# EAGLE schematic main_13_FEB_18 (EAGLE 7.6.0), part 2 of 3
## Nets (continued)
U_TRAP_2: IC159.15(D4)
U_TRAP_3: IC142.15(D4)
U_TRAP_4: IC129.15(D4)
U_TRAP_5: IC73.15(D4)
U_TRAP_6: IC34.15(D4)
U_TRAP_7: IC35.15(D4)
U_TRAP_8: IC36.15(D4)
U_TRAP_9: IC37.15(D4)
U_TRAP_10: IC38.15(D4)
U_TRAP_11: IC40.15(D4)
U_TRAP_12: IC41.15(D4)
U_TRAP_13: IC71.15(D4)
U_TRAP_14: IC20.15(D4)
U_TRAP_15: IC172.15(D4)
U_ZF: IC47.1(A:I0) IC126.2(1Q) IC127.2(A:I1) IC155.5(1C1)
U_ZF_IN_SRC: IC121.1(!A!/B)
UZF_AND_ALUZF: IC47.2(A:I1) IC119.3(B:I)
VCC: IC8.2(A:D) IC8.4(A:PRE) IC44.1(A:CLR) IC49.2(1A) IC56.5(1C1) IC163.2(A:D) IC163.4(A:PRE) IC164.2(A:D) IC164.4(A:PRE) IC168.2(A:D) IC168.4(A:PRE) IC174.2(A:D) IC174.4(A:PRE) IC187.2(A:D) IC187.4(A:PRE) IC188.2(A:D) IC188.4(A:PRE) IC204.4(A:PRE) IC221.2(A:D) IC221.4(A:PRE) IC222.6(G1) R1.2 R2.2 R3.2 R9.2
WR: IC60.5(Q2) IC69.13(B:A2)
XBUS0: IC2.18(Y1) IC9.18(Y1) IC25.9(B:Y1) IC27.9(B:Y1) IC103.18(Y1) IC104.18(Y1) IC105.9(B:Y1) IC107.9(B:Y1) IC109.9(B:Y1) IC111.9(B:Y1) IC113.18(Y1) IC114.18(Y1) IC116.18(Y1) IC117.18(Y1) IC122.18(Y1) IC125.18(Y1) IC140.18(Y1) IC145.18(Y1) IC154.18(Y1) IC181.18(A:Y1) IC210.18(Y1) IC244.9(B:Y1) IC245.18(Y1) RN1.1
XBUS1: IC2.17(Y2) IC9.17(Y2) IC25.7(B:Y2) IC27.7(B:Y2) IC105.7(B:Y2) IC107.7(B:Y2) IC109.7(B:Y2) IC111.7(B:Y2) IC113.17(Y2) IC114.17(Y2) IC116.17(Y2) IC117.17(Y2) IC122.17(Y2) IC125.17(Y2) IC145.17(Y2) IC154.17(Y2) IC181.16(A:Y2) IC245.17(Y2) RN1.2
XBUS2: IC2.16(Y3) IC9.16(Y3) IC25.5(B:Y3) IC27.5(B:Y3) IC105.5(B:Y3) IC107.5(B:Y3) IC109.5(B:Y3) IC111.5(B:Y3) IC113.16(Y3) IC114.16(Y3) IC116.16(Y3) IC117.16(Y3) IC122.16(Y3) IC125.16(Y3) IC145.16(Y3) IC154.16(Y3) IC181.14(A:Y3) IC245.16(Y3) RN1.3
XBUS3: IC2.15(Y4) IC9.15(Y4) IC25.3(B:Y4) IC27.3(B:Y4) IC105.3(B:Y4) IC107.3(B:Y4) IC109.3(B:Y4) IC111.3(B:Y4) IC113.15(Y4) IC114.15(Y4) IC116.15(Y4) IC117.15(Y4) IC122.15(Y4) IC125.15(Y4) IC145.15(Y4) IC154.15(Y4) IC181.12(A:Y4) IC244.3(B:Y4) IC245.15(Y4) RN1.4
XBUS4: IC24.9(B:Y1) IC26.9(B:Y1) IC106.9(B:Y1) IC108.9(B:Y1) IC110.9(B:Y1) IC112.9(B:Y1) IC116.14(Y5) IC125.14(Y5) IC154.14(Y5) IC176.18(A:Y1) IC245.14(Y5) IC247.9(B:Y1) RN1.5
XBUS5: IC24.7(B:Y2) IC26.7(B:Y2) IC106.7(B:Y2) IC108.7(B:Y2) IC110.7(B:Y2) IC112.7(B:Y2) IC116.13(Y6) IC125.13(Y6) IC154.13(Y6) IC176.16(A:Y2) IC245.13(Y6) RN1.6
XBUS6: IC24.5(B:Y3) IC26.5(B:Y3) IC106.5(B:Y3) IC108.5(B:Y3) IC110.5(B:Y3) IC112.5(B:Y3) IC113.12(Y7) IC114.12(Y7) IC115.12(Y7) IC116.12(Y7) IC125.12(Y7) IC154.12(Y7) IC176.14(A:Y3) IC245.12(Y7) RN1.7
XBUS7: IC2.11(Y8) IC3.11(Y8) IC9.11(Y8) IC24.3(B:Y4) IC26.3(B:Y4) IC80.4(B:I0) IC102.11(Y8) IC103.11(Y8) IC104.11(Y8) IC106.3(B:Y4) IC108.3(B:Y4) IC110.3(B:Y4) IC112.3(B:Y4) IC113.11(Y8) IC114.11(Y8) IC115.11(Y8) IC116.11(Y8) IC117.11(Y8) IC122.11(Y8) IC125.11(Y8) IC130.5(B:I1) IC140.11(Y8) IC145.11(Y8) IC146.11(Y8) IC154.11(Y8) IC176.12(A:Y4) IC210.11(Y8) IC245.11(Y8) IC247.3(B:Y4) RN1.8
XBUS8: IC146.18(Y1)
XBUS9: IC146.17(Y2)
XBUS10: IC146.16(Y3)
XBUS11: IC146.15(Y4)
XBUS12: IC171.18(Y1) IC215.18(Y1)
XBUS13: IC171.11(Y8) IC215.11(Y8)
XBUS14: IC259.18(Y1) IC260.18(Y1)
XBUS15: IC259.11(Y8) IC260.11(Y8)
XBUS16: IC89.18(A:Y1) IC91.18(A:Y1)
XBUS17: IC89.16(A:Y2) IC91.16(A:Y2)
XBUS18: IC89.14(A:Y3) IC91.14(A:Y3)
XBUS19: IC89.12(A:Y4) IC91.12(A:Y4)
XBUS20: IC90.18(A:Y1) IC92.18(A:Y1)
XBUS21: IC90.16(A:Y2) IC92.16(A:Y2)
XBUS22: IC90.14(A:Y3) IC92.14(A:Y3)
XBUS23: IC90.12(A:Y4) IC92.12(A:Y4)
XBUS24: IC14.1(B0) RN2.1
XBUS25: IC14.22(B1) RN2.2
XBUS26: IC14.20(B2) RN2.3
XBUS27: IC14.18(B3) RN2.4
XBUS28: IC11.12(A:Y4) IC15.1(B0) RN2.5
XBUS29: IC11.14(A:Y3) IC15.22(B1) RN2.6
XBUS30: IC11.16(A:Y2) IC15.20(B2) RN2.7
XBUS31: IC11.18(A:Y1) IC15.18(B3) RN2.8
XBUS32: IC102.18(Y1)
XBUS33: IC102.17(Y2)
XBUS34: IC102.16(Y3)
XBUS35: IC102.15(Y4)
XBUS36: IC263.18(Y1) IC264.18(Y1)
XBUS37: IC263.11(Y8) IC264.11(Y8)
XBUS38: IC252.18(Y1) IC253.18(Y1)
XBUS39: IC252.11(Y8) IC253.11(Y8)
XBUS40: IC3.18(Y1)
XBUS41: IC3.17(Y2)
XBUS42: IC3.16(Y3)
XBUS43: IC3.15(Y4)
XBUS44: IC266.18(Y1) IC267.18(Y1)
XBUS45: IC266.11(Y8) IC267.11(Y8)
XBUS46: IC298.18(A:Y1)
XBUS47: IC298.16(A:Y2)
XBUS48: IC115.18(Y1)
XBUS49: IC115.17(Y2)
XBUS50: IC115.16(Y3)
XBUS51: IC115.15(Y4)
XBUS52: IC298.14(A:Y3)
XBUS53: IC298.12(A:Y4)
XBUS54: IC297.18(A:Y1)
XBUS55: IC297.16(A:Y2)
XBUS56: IC15.19(A3) RN3.1
XBUS57: IC15.21(A2) RN3.2
XBUS58: IC15.23(A1) RN3.3
XBUS59: IC15.2(A0) RN3.4
XBUS60: IC14.19(A3) RN3.5
XBUS61: IC14.21(A2) RN3.6
XBUS62: IC14.23(A1) RN3.7
XBUS63: IC14.2(A0) RN3.8
XBUS64: IC297.14(A:Y3)
XBUS65: IC297.12(A:Y4)
XBUS66: IC289.12(A:Y4)
XBUS67: IC289.14(A:Y3)
XBUS68: IC289.16(A:Y2)
XBUS69: IC289.18(A:Y1)
YBUS0: IC19.18(Y1) IC182.18(A:Y1)
YBUS1: IC19.17(Y2) IC182.16(A:Y2)
YBUS2: IC19.16(Y3) IC182.14(A:Y3)
YBUS3: IC19.15(Y4) IC182.12(A:Y4)
YBUS4: IC19.14(Y5) IC183.18(A:Y1)
YBUS5: IC183.16(A:Y2)
YBUS6: IC183.14(A:Y3)
YBUS7: IC19.11(Y8) IC130.4(B:I0) IC183.12(A:Y4)
YBUS8: IC299.18(A:Y1)
YBUS9: IC299.16(A:Y2)
YBUS10: IC299.14(A:Y3)
YBUS11: IC299.12(A:Y4)
YBUS12: IC300.18(A:Y1)
YBUS13: IC300.16(A:Y2)
YBUS14: IC300.14(A:Y3)
YBUS15: IC300.12(A:Y4)
YBUS16: IC211.18(A:Y1) IC213.18(A:Y1)
YBUS17: IC211.16(A:Y2) IC213.16(A:Y2)
YBUS18: IC211.14(A:Y3) IC213.14(A:Y3)
YBUS19: IC211.12(A:Y4) IC213.12(A:Y4)
YBUS20: IC212.18(A:Y1) IC214.18(A:Y1)
YBUS21: IC212.16(A:Y2) IC214.16(A:Y2)
YBUS22: IC212.14(A:Y3) IC214.14(A:Y3)
YBUS23: IC212.12(A:Y4) IC214.12(A:Y4)
YBUS40: IC229.18(A:Y1) IC231.18(A:Y1)
YBUS41: IC229.16(A:Y2) IC231.16(A:Y2)
YBUS42: IC229.14(A:Y3) IC231.14(A:Y3)
YBUS43: IC229.12(A:Y4) IC231.12(A:Y4)
YBUS44: IC230.18(A:Y1) IC232.18(A:Y1)
YBUS45: IC230.16(A:Y2) IC232.16(A:Y2)
YBUS46: IC230.14(A:Y3) IC232.14(A:Y3)
YBUS47: IC230.12(A:Y4) IC232.12(A:Y4)
YBUS48: IC235.18(A:Y1) IC237.18(A:Y1)
YBUS49: IC235.16(A:Y2) IC237.16(A:Y2)
YBUS50: IC235.14(A:Y3) IC237.14(A:Y3)
YBUS51: IC235.12(A:Y4) IC237.12(A:Y4)
YBUS52: IC236.18(A:Y1) IC238.18(A:Y1)
YBUS53: IC236.16(A:Y2) IC238.16(A:Y2)
YBUS54: IC236.14(A:Y3) IC238.14(A:Y3)
YBUS55: IC236.12(A:Y4) IC238.12(A:Y4)
ZBUFF0_16: IC86.3(1D) IC88.3(1D)
ZBUFF0_17: IC86.4(2D) IC88.4(2D)
ZBUFF0_18: IC86.7(3D) IC88.7(3D)
ZBUFF0_19: IC86.8(4D) IC88.8(4D)
ZBUFF0_20: IC86.13(5D) IC88.13(5D)
ZBUFF0_21: IC88.14(6D)
ZBUFF0_22: IC86.14(6D) IC86.17(7D) IC88.17(7D)
ZBUFF0_23: IC86.18(8D) IC88.18(8D)
ZBUFF0_24: IC16.3(1D) IC17.3(1D)
ZBUFF0_25: IC16.4(2D) IC17.4(2D)
ZBUFF0_26: IC16.7(3D) IC17.7(3D)
ZBUFF0_27: IC16.8(4D) IC17.8(4D)
ZBUFF0_28: IC16.13(5D) IC17.13(5D)
ZBUFF0_29: IC16.14(6D) IC17.14(6D)
ZBUFF0_30: IC16.17(7D) IC17.17(7D)
ZBUFF0_31: IC16.18(8D) IC17.18(8D)
ZBUFF0_56: IC233.3(1D) IC234.3(1D)
ZBUFF0_57: IC233.4(2D) IC234.4(2D)
ZBUFF0_58: IC233.7(3D) IC234.7(3D)
ZBUFF0_59: IC233.8(4D) IC234.8(4D)
ZBUFF0_60: IC233.13(5D) IC234.13(5D)
ZBUFF0_61: IC233.14(6D) IC234.14(6D)
ZBUFF0_62: IC233.17(7D) IC234.17(7D)
ZBUFF0_63: IC233.18(8D) IC234.18(8D)
ZBUFF0_64: IC239.3(1D) IC240.3(1D)
ZBUFF0_65: IC239.4(2D) IC240.4(2D)
ZBUFF0_66: IC239.7(3D) IC240.7(3D)
ZBUFF0_67: IC239.8(4D) IC240.8(4D)
ZBUFF0_68: IC239.13(5D) IC240.13(5D)
ZBUFF0_69: IC239.14(6D) IC240.14(6D)
ZBUFF0_70: IC239.17(7D) IC240.17(7D)
ZBUFF0_71: IC239.18(8D) IC240.18(8D)
ZBUFF1_0: IC4.3(1D) IC5.3(1D) IC98.3(1D) IC99.3(1D)
ZBUFF1_1: IC4.4(2D) IC5.4(2D) IC98.4(2D) IC99.4(2D)
ZBUFF1_2: IC4.7(3D) IC5.7(3D) IC98.7(3D) IC99.7(3D)
ZBUFF1_3: IC4.8(4D) IC5.8(4D) IC98.8(4D) IC99.8(4D)
ZBUFF1_4: IC4.13(5D) IC5.13(5D) IC98.13(5D) IC99.13(5D)
ZBUFF1_5: IC4.14(6D) IC5.14(6D) IC98.14(6D) IC99.14(6D)
ZBUFF1_6: IC4.17(7D) IC5.17(7D) IC98.17(7D) IC99.17(7D)
ZBUFF1_7: IC4.18(8D) IC5.18(8D) IC98.18(8D) IC99.18(8D)
ZBUFF1_8: IC173.3(1D) IC205.3(1D)
ZBUFF1_9: IC173.4(2D) IC205.4(2D)
ZBUFF1_10: IC173.7(3D) IC205.7(3D)
ZBUFF1_11: IC173.8(4D) IC205.8(4D)
ZBUFF1_12: IC173.13(5D) IC205.13(5D)
ZBUFF1_13: IC173.14(6D) IC205.14(6D)
ZBUFF1_14: IC173.17(7D) IC205.17(7D)
ZBUFF1_15: IC173.18(8D) IC205.18(8D)
ZBUFF1_16: IC165.3(1D) IC166.3(1D)
ZBUFF1_17: IC165.4(2D) IC166.4(2D)
ZBUFF1_18: IC165.7(3D) IC166.7(3D)
ZBUFF1_19: IC165.8(4D) IC166.8(4D)
ZBUFF1_20: IC165.13(5D) IC166.13(5D)
ZBUFF1_21: IC165.14(6D) IC166.14(6D)
ZBUFF1_22: IC165.17(7D) IC166.17(7D)
ZBUFF1_23: IC165.18(8D) IC166.18(8D)
ZBUFF1_24: IC217.3(1D) IC246.3(1D)
ZBUFF1_25: IC217.4(2D) IC246.4(2D)
ZBUFF1_26: IC217.7(3D) IC246.7(3D)
ZBUFF1_27: IC217.8(4D) IC246.8(4D)
ZBUFF1_28: IC217.13(5D) IC246.13(5D)
ZBUFF1_29: IC217.14(6D) IC246.14(6D)
ZBUFF1_30: IC217.17(7D) IC246.17(7D)
ZBUFF1_31: IC217.18(8D) IC246.18(8D)
ZBUFF1_32: IC261.3(1D) IC262.3(1D)
ZBUFF1_33: IC261.4(2D) IC262.4(2D)
ZBUFF1_34: IC261.7(3D) IC262.7(3D)
ZBUFF1_35: IC261.8(4D) IC262.8(4D)
ZBUFF1_36: IC261.13(5D) IC262.13(5D)
ZBUFF1_37: IC261.14(6D) IC262.14(6D)
ZBUFF1_38: IC261.17(7D) IC262.17(7D)
ZBUFF1_39: IC261.18(8D) IC262.18(8D)
ZBUFF1_40: IC202.3(1D) IC251.3(1D)
ZBUFF1_41: IC202.4(2D) IC251.4(2D)
ZBUFF1_42: IC202.7(3D) IC251.7(3D)
ZBUFF1_43: IC202.8(4D) IC251.8(4D)
ZBUFF1_44: IC202.13(5D) IC251.13(5D)
ZBUFF1_45: IC202.14(6D) IC251.14(6D)
ZBUFF1_46: IC202.17(7D) IC251.17(7D)
ZBUFF1_47: IC202.18(8D) IC251.18(8D)
ZBUFF1_48: IC254.3(1D) IC265.3(1D)
ZBUFF1_49: IC254.4(2D) IC265.4(2D)
ZBUFF1_50: IC254.7(3D) IC265.7(3D)
ZBUFF1_51: IC254.8(4D) IC265.8(4D)
ZBUFF1_52: IC254.13(5D) IC265.13(5D)
ZBUFF1_53: IC254.14(6D) IC265.14(6D)
ZBUFF1_54: IC254.17(7D) IC265.17(7D)
ZBUFF1_55: IC254.18(8D) IC265.18(8D)
ZBUFF2_0: IC1.3(1D) IC23.14(4A) IC100.3(1D) IC101.3(1D)
ZBUFF2_1: IC1.4(2D) IC23.11(3A) IC100.4(2D) IC101.4(2D)
ZBUFF2_2: IC1.7(3D) IC23.5(2A) IC100.7(3D) IC101.7(3D)
ZBUFF2_3: IC1.8(4D) IC23.2(1A) IC100.8(4D) IC101.8(4D)
ZBUFF2_4: IC1.13(5D) IC22.14(4A) IC100.13(5D) IC101.13(5D)
ZBUFF2_5: IC1.14(6D) IC22.11(3A) IC100.14(6D) IC101.14(6D)
ZBUFF2_6: IC1.17(7D) IC22.5(2A) IC100.17(7D) IC101.17(7D)
ZBUFF2_7: IC22.2(1A) IC100.18(8D) IC101.18(8D)
ZBUFF2_16: IC123.3(1D)
ZBUFF2_17: IC123.4(2D)
ZBUFF2_18: IC123.7(3D)
ZBUFF2_19: IC123.8(4D)
ZBUFF2_20: IC123.13(5D)
ZBUFF2_21: IC123.14(6D)
ZBUFF2_22: IC123.17(7D)
ZBUFF2_23: IC153.3(1D)
ZBUFF2_24: IC153.4(2D)
ZBUFF2_25: IC153.7(3D)
ZBUFF2_26: IC153.8(4D)
ZBUFF2_27: IC153.13(5D)
ZBUFF2_28: IC153.14(6D)
ZBUFF2_29: IC153.17(7D)
ZBUFF2_30: IC153.18(8D)
ZBUFF2_31: IC185.3(1D)
ZBUFF2_32: IC185.4(2D)
ZBUFF2_33: IC185.7(3D)
ZBUFF2_34: IC185.8(4D)
ZBUFF2_35: IC185.13(5D)
ZBUFF2_36: IC185.14(6D)
ZBUFF2_37: IC185.17(7D)
ZBUFF2_38: IC185.18(8D)
ZBUS0: IC6.3(1D) IC7.3(1D) IC48.3(1D) IC96.2(1A) IC97.2(1A) IC144.14(D1) IC175.4(B:I0) IC184.3(1D) IC189.3(1D) IC197.1(A:I0) IC216.3(1D) IC241.3(1C3) IC248.14(D1) RN5.1
ZBUS1: IC96.5(2A) IC97.5(2A) IC144.13(D2) IC175.5(B:I1) IC184.4(2D) IC197.2(A:I1) IC216.4(2D) IC243.3(1C3) IC248.13(D2) RN5.2
ZBUS2: IC96.11(3A) IC97.11(3A) IC144.12(D3) IC177.5(B:I1) IC184.7(3D) IC197.3(A:I2) IC216.7(3D) IC248.12(D3) IC255.3(1C3) RN5.3
ZBUS3: IC96.14(4A) IC97.14(4A) IC144.11(D4) IC184.8(4D) IC192.5(B:I1) IC197.12(A:I3) IC216.8(4D) IC248.11(D4) IC256.3(1C3) RN5.4
ZBUS4: IC94.2(1A) IC95.2(1A) IC128.14(D1) IC184.13(5D) IC193.5(B:I1) IC197.13(A:I4) IC208.3(1C3) IC216.13(5D) IC249.14(D1) RN5.5
ZBUS5: IC94.5(2A) IC95.5(2A) IC128.13(D2) IC184.14(6D) IC194.5(B:I1) IC199.2(A:I1) IC216.14(6D) IC249.13(D2) RN5.6
ZBUS6: IC94.11(3A) IC95.11(3A) IC128.12(D3) IC184.17(7D) IC199.3(A:I2) IC200.5(B:I1) IC216.17(7D) IC249.12(D3) RN5.7
ZBUS7: IC6.18(8D) IC7.18(8D) IC48.18(8D) IC80.5(B:I1) IC94.14(4A) IC95.14(4A) IC128.11(D4) IC184.18(8D) IC189.18(8D) IC199.12(A:I3) IC209.5(B:I1) IC216.18(8D) IC249.11(D4) IC255.5(1C1) RN5.8
ZF: IC120.2(A:I1) IC122.2(A1) IC155.6(1C0) IC227.2(Q1) IC241.6(1C0)
ZF_FROM_ALU: IC120.1(A:I0) IC121.2(1A) IC124.1(A:I0) IC127.1(A:I0) IC155.4(1C2) IC199.5(A:O) IC241.5(1C1)
ZF_IN_SRC_0: IC241.14(A)
ZF_IN_SRC_1: IC241.2(B)
~CLK: IC32.11(CLK) IC33.11(CLK)
~RST: IC32.1(CLR) IC33.1(CLR) IC44.4(A:PRE) IC54.4(B:O) IC162.1(CLR) IC195.1(A:I0) IC204.1(A:CLR) IC207.2(A:I1) IC218.1(A:I0) IC219.1(A:I0) IC220.2(A:I1) IC223.2(A:I1) IC224.2(A:I1) IC225.2(A:I1) IC227.1(CLR)
Unconnected: IC1.11(CLK) IC1.18(8D) IC2.12(Y7) IC2.13(Y6) IC2.14(Y5) IC3.12(Y7) IC3.13(Y6) IC3.14(Y5) IC4.11(CLK) IC5.11(CLK) IC6.4(2D) IC6.7(3D) IC6.8(4D) IC6.11(CLK) IC6.13(5D) IC6.14(6D) IC6.17(7D) IC7.4(2D) IC7.7(3D) IC7.8(4D) IC7.13(5D) IC7.14(6D) IC7.17(7D) IC8.6(A:!Q) IC8.8(B:!Q) IC8.9(B:Q) IC8.10(B:PRE) IC8.11(B:CLK) IC8.12(B:D) IC8.13(B:CLR) IC9.12(Y7) IC9.13(Y6) IC9.14(Y5) IC10.3(B:Y4) IC10.5(B:Y3) IC10.7(B:Y2) IC10.9(B:Y1) IC10.11(B:A1) IC10.13(B:A2) IC10.15(B:A3) IC10.17(B:A4) IC10.19(B:G) IC11.3(B:Y4) IC11.5(B:Y3) IC11.7(B:Y2) IC11.9(B:Y1) IC11.11(B:A1) IC11.13(B:A2) IC11.15(B:A3) IC11.17(B:A4) IC11.19(B:G) IC12.3(B:Y4) IC12.5(B:Y3) IC12.7(B:Y2) IC12.9(B:Y1) IC12.11(B:A1) IC12.13(B:A2) IC12.15(B:A3) IC12.17(B:A4) IC12.19(B:G) IC13.3(B:Y4) IC13.5(B:Y3) IC13.7(B:Y2) IC13.9(B:Y1) IC13.11(B:A1) IC13.13(B:A2) IC13.15(B:A3) IC13.17(B:A4) IC13.19(B:G) IC14.14(A=B) IC14.15(P) IC14.17(G) IC15.14(A=B) IC15.15(P) IC15.17(G) IC16.11(CLK) IC17.11(CLK) IC18.1(A:I0) IC18.2(A:I1) IC18.3(A:O) IC18.8(C:O) IC18.9(C:I0) IC18.10(C:I1) IC18.11(D:O) IC18.12(D:I0) IC18.13(D:I1) IC19.2(A1) IC19.3(A2) IC19.4(A3) IC19.5(A4) IC19.6(A5) IC19.7(A6) IC19.8(A7) IC19.9(A8) IC19.12(Y7) IC19.13(Y6) IC20.6(W) IC20.7(G) IC20.9(C) IC20.10(B) IC20.11(A) IC20.12(D7) IC20.13(D6) IC21.11(CLK) IC24.1(A:G) IC24.2(A:A1) IC24.4(A:A2) IC24.6(A:A3) IC24.8(A:A4) IC24.12(A:Y4) IC24.14(A:Y3) IC24.16(A:Y2) IC24.18(A:Y1) IC25.1(A:G) IC25.2(A:A1) IC25.4(A:A2) IC25.6(A:A3) IC25.8(A:A4) IC25.12(A:Y4) IC25.14(A:Y3) IC25.16(A:Y2) IC25.18(A:Y1) IC26.1(A:G) IC26.2(A:A1) IC26.4(A:A2) IC26.6(A:A3) IC26.8(A:A4) IC26.12(A:Y4) IC26.14(A:Y3) IC26.16(A:Y2) IC26.18(A:Y1) IC27.1(A:G) IC27.2(A:A1) IC27.4(A:A2) IC27.6(A:A3) IC27.8(A:A4) IC27.12(A:Y4) IC27.14(A:Y3) IC27.16(A:Y2) IC27.18(A:Y1) IC28.6(A5) IC28.7(A6) IC28.8(A7) IC28.9(A8) IC28.11(Y8) IC28.12(Y7) IC28.13(Y6) IC28.14(Y5) IC30.3(B:Y4) IC30.5(B:Y3) IC30.7(B:Y2) IC30.9(B:Y1) IC30.11(B:A1) IC30.13(B:A2) IC30.15(B:A3) IC30.17(B:A4) IC30.19(B:G) IC31.3(B:Y4) IC31.5(B:Y3) IC31.7(B:Y2) IC31.9(B:Y1) IC31.11(B:A1) IC31.13(B:A2) IC31.15(B:A3) IC31.17(B:A4) IC31.19(B:G) IC34.6(W) IC34.7(G) IC34.9(C) IC34.10(B) IC34.11(A) IC34.12(D7) IC34.13(D6) IC35.6(W) IC35.7(G) IC35.9(C) IC35.10(B) IC35.11(A) IC35.12(D7) IC35.13(D6) IC36.6(W) IC36.7(G) IC36.9(C) IC36.10(B) IC36.11(A) IC36.12(D7) IC36.13(D6) IC37.6(W) IC37.7(G) IC37.9(C) IC37.10(B) IC37.11(A) IC37.12(D7) IC37.13(D6) IC38.6(W) IC38.7(G) IC38.9(C) IC38.10(B) IC38.11(A) IC38.12(D7) IC38.13(D6) IC39.4(B:I0) IC39.5(B:I1) IC39.6(B:O) IC39.8(C:O) IC39.9(C:I0) IC39.10(C:I1) IC39.11(D:O) IC39.12(D:I0) IC39.13(D:I1) IC40.6(W) IC40.7(G) IC40.9(C) IC40.10(B) IC40.11(A) IC40.12(D7) IC40.13(D6) IC41.6(W) IC41.7(G) IC41.9(C) IC41.10(B) IC41.11(A) IC41.12(D7) IC41.13(D6) IC42.4(B:I0) IC42.5(B:I1) IC42.6(B:O) IC42.8(C:O) IC42.9(C:I0) IC42.10(C:I1) IC42.11(D:O) IC42.12(D:I0) IC42.13(D:I1) IC43.1(A:I) IC43.2(A:O) IC43.5(C:I) IC43.6(C:O) IC43.8(D:O) IC43.9(D:I) IC43.10(E:O) IC43.11(E:I) IC43.12(F:O) IC43.13(F:I) IC44.6(A:!Q) IC44.8(B:!Q) IC44.9(B:Q) IC44.10(B:PRE) IC44.11(B:CLK) IC44.12(B:D) IC44.13(B:CLR) IC45.4(B:I0) IC45.5(B:I1) IC45.6(B:O) IC45.8(C:O) IC45.9(C:I0) IC45.10(C:I1) IC45.11(D:O) IC45.12(D:I0) IC45.13(D:I1) IC46.1(A:I0) IC46.2(A:I1) IC46.3(A:O) IC46.8(C:O) IC46.9(C:I0) IC46.10(C:I1) IC46.11(D:O) IC46.12(D:I0) IC46.13(D:I1) IC47.4(B:I0) IC47.5(B:I1) IC47.6(B:O) IC47.8(C:O) IC47.9(C:I0) IC47.10(C:I1) IC47.11(D:O) IC47.12(D:I0) IC47.13(D:I1) IC48.4(2D) IC48.7(3D) IC48.8(4D) IC48.11(CLK) IC48.13(5D) IC48.14(6D) IC48.17(7D) IC50.1(S2) IC50.10(S4) IC50.13(S3) IC51.1(S2) IC51.4(S1) IC51.10(S4) IC51.13(S3) IC52.1(S2) IC52.4(S1) IC52.10(S4) IC52.13(S3) IC53.4(S1) IC53.9(C4) IC53.10(S4) IC53.13(S3) IC54.1(A:I) IC54.2(A:O) IC54.5(C:I) IC54.6(C:O) IC54.8(D:O) IC54.9(D:I) IC54.10(E:O) IC54.11(E:I) IC54.12(F:O) IC54.13(F:I) IC56.9(2Y) IC56.10(2C0) IC56.11(2C1) IC56.12(2C2) IC56.13(2C3) IC57.5(C:I) IC57.6(C:O) IC57.8(D:O) IC57.9(D:I) IC57.10(E:O) IC57.11(E:I) IC57.12(F:O) IC57.13(F:I) IC58.4(B:I0) IC58.5(B:I1) IC58.6(B:O) IC58.8(C:O) IC58.9(C:I0) IC58.10(C:I1) IC58.11(D:O) IC58.12(D:I0) IC58.13(D:I1) IC59.3(B:I) IC59.4(B:O) IC59.5(C:I) IC59.6(C:O) IC59.8(D:O) IC59.9(D:I) IC59.10(E:O) IC59.11(E:I) IC59.12(F:O) IC59.13(F:I) IC60.1(CLR) IC60.9(Q4) IC60.12(Q5) IC60.15(Q6) IC60.16(Q7) IC60.19(Q8) IC61.1(CLR) IC61.2(Q1) IC61.5(Q2) IC61.6(Q3) IC61.9(Q4) IC61.12(Q5) IC61.15(Q6) IC61.16(Q7) IC61.19(Q8) IC62.1(CLR) IC62.2(Q1) IC62.5(Q2) IC62.6(Q3) IC62.9(Q4) IC62.12(Q5) IC62.15(Q6) IC62.16(Q7) IC62.19(Q8) IC64.3(B:I0) IC64.4(B:I1) IC64.5(B:I2) IC64.6(B:O) IC64.8(C:O) IC64.9(C:I0) IC64.10(C:I1) IC64.11(C:I2) IC65.4(B:O) IC65.5(B:I0) IC65.6(B:I1) IC65.8(C:I0) IC65.9(C:I1) IC65.10(C:O) IC65.11(D:I0) IC65.12(D:I1) IC65.13(D:O) IC66.4(B:O) IC66.5(B:I0) IC66.6(B:I1) IC66.8(C:I0) IC66.9(C:I1) IC66.10(C:O) IC66.11(D:I0) IC66.12(D:I1) IC66.13(D:O) IC67.1(A:I0) IC67.2(A:I1) IC67.3(A:O) IC67.8(C:O) IC67.9(C:I0) IC67.10(C:I1) IC67.11(D:O) IC67.12(D:I0) IC67.13(D:I1) IC68.9(3Y) IC68.12(4Y) IC69.1(A:G) IC69.2(A:A1) IC69.3(B:Y4) IC69.4(A:A2) IC69.6(A:A3) IC69.8(A:A4) IC69.12(A:Y4) IC69.14(A:Y3) IC69.16(A:Y2) IC69.18(A:Y1) IC70.6(W) IC71.6(W) IC71.7(G) IC71.9(C) IC71.10(B) IC71.11(A) IC71.12(D7) IC71.13(D6) IC72.1(A:I0) IC72.2(A:I1) IC72.3(A:O) IC72.8(C:O) IC72.9(C:I0) IC72.10(C:I1) IC72.11(D:O) IC72.12(D:I0) IC72.13(D:I1) IC73.6(W) IC73.7(G) IC73.9(C) IC73.10(B) IC73.11(A) IC73.12(D7) IC73.13(D6) IC74.1(A:I0) IC74.2(A:I1) IC74.3(A:O) IC74.8(C:O) IC74.9(C:I0) IC74.10(C:I1) IC74.11(D:O) IC74.12(D:I0) IC74.13(D:I1) IC75.2(Q1) IC75.5(Q2) IC75.6(Q3) IC75.9(Q4) IC75.12(Q5) IC75.15(Q6) IC75.16(Q7) IC75.19(Q8) IC76.2(Q1) IC77.2(Q1) IC78.2(Q1) IC78.5(Q2) IC78.6(Q3) IC78.9(Q4) IC78.12(Q5) IC78.15(Q6) IC78.16(Q7) IC78.19(Q8) IC79.2(Q1) IC79.5(Q2) IC79.6(Q3) IC79.9(Q4) IC79.12(Q5) IC79.15(Q6) IC79.16(Q7) IC79.19(Q8) IC80.1(A:I0) IC80.2(A:I1) IC80.3(A:O) IC80.8(C:O) IC80.9(C:I0) IC80.10(C:I1) IC80.11(D:O) IC80.12(D:I0) IC80.13(D:I1) IC81.1(A:I0) IC81.2(A:I1) IC81.3(A:O) IC81.8(C:O) IC81.9(C:I0) IC81.10(C:I1) IC81.11(D:O) IC81.12(D:I0) IC81.13(D:I1) IC82.11(CLK) IC83.1(A:I) IC83.2(A:O) IC83.5(C:I) IC83.6(C:O) IC83.8(D:O) IC83.9(D:I) IC83.10(E:O) IC83.11(E:I) IC83.12(F:O) IC83.13(F:I) IC84.1(A:I) IC84.2(A:O) IC84.5(C:I) IC84.6(C:O) IC84.8(D:O) IC84.9(D:I) IC84.10(E:O) IC84.11(E:I) IC84.12(F:O) IC84.13(F:I) IC85.3(B:I0) IC85.4(B:I1) IC85.5(B:I2) IC85.6(B:O) IC85.8(C:O) IC85.9(C:I0) IC85.10(C:I1) IC85.11(C:I2) IC86.11(CLK) IC87.2(A:S1) IC87.5(C:R) IC87.6(C:S) IC87.7(C:Q) IC87.9(B:Q) IC87.10(B:R) IC87.11(B:S1) IC87.12(B:S2) IC87.13(D:Q) IC87.14(D:R) IC87.15(D:S) IC88.11(CLK) IC89.3(B:Y4) IC89.5(B:Y3) IC89.7(B:Y2) IC89.9(B:Y1) IC89.11(B:A1) IC89.13(B:A2) IC89.15(B:A3) IC89.17(B:A4) IC89.19(B:G) IC90.3(B:Y4) IC90.5(B:Y3) IC90.7(B:Y2) IC90.9(B:Y1) IC90.11(B:A1) IC90.13(B:A2) IC90.15(B:A3) IC90.17(B:A4) IC90.19(B:G) IC91.3(B:Y4) IC91.5(B:Y3) IC91.7(B:Y2) IC91.9(B:Y1) IC91.11(B:A1) IC91.13(B:A2) IC91.15(B:A3) IC91.17(B:A4) IC91.19(B:G) IC92.3(B:Y4) IC92.5(B:Y3) IC92.7(B:Y2) IC92.9(B:Y1) IC92.11(B:A1) IC92.13(B:A2) IC92.15(B:A3) IC92.17(B:A4) IC92.19(B:G) IC93.11(CLK) IC98.11(CLK) IC99.11(CLK) IC100.11(CLK) IC101.11(CLK) IC102.12(Y7) IC102.13(Y6) IC102.14(Y5) IC103.12(Y7) IC103.13(Y6) IC103.14(Y5) IC103.15(Y4) IC103.16(Y3) IC103.17(Y2) IC104.12(Y7) IC104.13(Y6) IC104.14(Y5) IC104.15(Y4) IC104.16(Y3) IC104.17(Y2) IC105.1(A:G) IC105.2(A:A1) IC105.4(A:A2) IC105.6(A:A3) IC105.8(A:A4) IC105.12(A:Y4) IC105.14(A:Y3) IC105.16(A:Y2) IC105.18(A:Y1) IC106.1(A:G) IC106.2(A:A1) IC106.4(A:A2) IC106.6(A:A3) IC106.8(A:A4) IC106.12(A:Y4) IC106.14(A:Y3) IC106.16(A:Y2) IC106.18(A:Y1) IC107.1(A:G) IC107.2(A:A1) IC107.4(A:A2) IC107.6(A:A3) IC107.8(A:A4) IC107.12(A:Y4) IC107.14(A:Y3) IC107.16(A:Y2) IC107.18(A:Y1) IC108.1(A:G) IC108.2(A:A1) IC108.4(A:A2) IC108.6(A:A3) IC108.8(A:A4) IC108.12(A:Y4) IC108.14(A:Y3) IC108.16(A:Y2) IC108.18(A:Y1) IC109.1(A:G) IC109.2(A:A1) IC109.4(A:A2) IC109.6(A:A3) IC109.8(A:A4) IC109.12(A:Y4) IC109.14(A:Y3) IC109.16(A:Y2) IC109.18(A:Y1) IC110.1(A:G) IC110.2(A:A1) IC110.4(A:A2) IC110.6(A:A3) IC110.8(A:A4) IC110.12(A:Y4) IC110.14(A:Y3) IC110.16(A:Y2) IC110.18(A:Y1) IC111.1(A:G) IC111.2(A:A1) IC111.4(A:A2) IC111.6(A:A3) IC111.8(A:A4) IC111.12(A:Y4) IC111.14(A:Y3) IC111.16(A:Y2) IC111.18(A:Y1) IC112.1(A:G) IC112.2(A:A1) IC112.4(A:A2) IC112.6(A:A3) IC112.8(A:A4) IC112.12(A:Y4) IC112.14(A:Y3) IC112.16(A:Y2) IC112.18(A:Y1) IC113.13(Y6) IC113.14(Y5) IC113.19(G2) IC114.13(Y6) IC114.14(Y5) IC114.19(G2) IC115.13(Y6) IC115.14(Y5) IC117.12(Y7) IC117.13(Y6) IC117.14(Y5) IC118.6(3Q) IC118.7(3D) IC118.8(4D) IC118.9(4Q) IC118.11(CLK) IC118.12(5Q) IC118.13(5D) IC118.14(6D) IC118.15(6Q) IC118.16(7Q) IC118.17(7D) IC118.18(8D) IC118.19(8Q) IC119.1(A:I) IC119.2(A:O) IC119.5(C:I) IC119.6(C:O) IC119.8(D:O) IC119.9(D:I) IC119.10(E:O) IC119.11(E:I) IC119.12(F:O) IC119.13(F:I) IC120.4(B:I0) IC120.5(B:I1) IC120.6(B:O) IC120.8(C:O) IC120.9(C:I0) IC120.10(C:I1) IC120.11(D:O) IC120.12(D:I0) IC120.13(D:I1) IC121.4(1Y) IC121.5(2A) IC121.6(2B) IC121.7(2Y) IC121.9(3Y) IC121.10(3B) IC121.11(3A) IC121.12(4Y) IC121.13(4B) IC121.14(4A) IC122.12(Y7) IC122.13(Y6) IC122.14(Y5) IC123.11(CLK) IC123.18(8D) IC124.4(B:I0) IC124.5(B:I1) IC124.6(B:O) IC124.8(C:O) IC124.9(C:I0) IC124.10(C:I1) IC124.11(D:O) IC124.12(D:I0) IC124.13(D:I1) IC126.11(CLK) IC126.12(5Q) IC126.13(5D) IC126.14(6D) IC126.15(6Q) IC126.16(7Q) IC126.17(7D) IC126.18(8D) IC126.19(8Q) IC127.4(B:I0) IC127.5(B:I1) IC127.6(B:O) IC127.8(C:O) IC127.9(C:I0) IC127.10(C:I1) IC127.11(D:O) IC127.12(D:I0) IC127.13(D:I1) IC129.6(W) IC129.7(G) IC129.9(C) IC129.10(B) IC129.11(A) IC129.12(D7) IC129.13(D6) IC130.1(A:I0) IC130.2(A:I1) IC130.3(A:O) IC130.8(C:O) IC130.9(C:I0) IC130.10(C:I1) IC130.11(D:O) IC130.12(D:I0) IC130.13(D:I1) IC131.4(B:O) IC131.5(B:I0) IC131.6(B:I1) IC131.8(C:I0) IC131.9(C:I1) IC131.10(C:O) IC131.11(D:I0) IC131.12(D:I1) IC131.13(D:O) IC132.3(B:I0) IC132.4(B:I1) IC132.5(B:I2) IC132.6(B:O) IC132.8(C:O) IC132.9(C:I0) IC132.10(C:I1) IC132.11(C:I2) IC133.3(A:O) IC133.4(B:I0) IC133.5(B:I1) IC133.6(B:O) IC133.8(C:O) IC133.9(C:I0) IC133.10(C:I1) IC133.11(D:O) IC133.12(D:I0) IC133.13(D:I1) IC134.2(Q1) IC134.5(Q2) IC134.6(Q3) IC134.9(Q4) IC134.12(Q5) IC134.15(Q6) IC134.16(Q7) IC134.19(Q8) IC135.2(Q1) IC135.5(Q2) IC135.6(Q3) IC135.9(Q4) IC135.12(Q5) IC135.15(Q6) IC135.16(Q7) IC135.19(Q8) IC136.2(Q1) IC136.5(Q2) IC136.6(Q3) IC136.9(Q4) IC136.12(Q5) IC136.15(Q6) IC136.16(Q7) IC136.19(Q8) IC137.2(Q1) IC137.5(Q2) IC137.6(Q3) IC137.9(Q4) IC137.12(Q5) IC137.15(Q6) IC137.16(Q7) IC137.19(Q8) IC138.3(B:I0) IC138.4(B:I1) IC138.5(B:I2) IC138.6(B:O) IC138.8(C:O) IC138.9(C:I0) IC138.10(C:I1) IC138.11(C:I2) IC139.4(Q2) IC139.5(Q3) IC139.6(Q4) IC139.11(D4) IC139.12(D3) IC139.13(D2) IC140.12(Y7) IC140.13(Y6) IC140.14(Y5) IC140.15(Y4) IC140.16(Y3) IC140.17(Y2) IC141.8(C:O) IC141.9(C:I0) IC141.10(C:I1) IC141.11(C:I2) IC142.6(W) IC142.7(G) IC142.9(C) IC142.10(B) IC142.11(A) IC142.12(D7) IC142.13(D6) IC143.4(B:I0) IC143.5(B:I1) IC143.6(B:O) IC143.8(C:O) IC143.9(C:I0) IC143.10(C:I1) IC143.11(D:O) IC143.12(D:I0) IC143.13(D:I1) IC145.12(Y7) IC145.13(Y6) IC145.14(Y5) IC146.12(Y7) IC146.13(Y6) IC146.14(Y5) IC147.1(A:I0) IC147.2(A:I1) IC147.3(A:O) IC147.8(C:O) IC147.9(C:I0) IC147.10(C:I1) IC147.11(D:O) IC147.12(D:I0) IC147.13(D:I1) IC148.4(B:I0) IC148.5(B:I1) IC148.6(B:O) IC148.8(C:O) IC148.9(C:I0) IC148.10(C:I1) IC148.11(D:O) IC148.12(D:I0) IC148.13(D:I1) IC149.1(A:I) IC149.2(A:O) IC149.5(C:I) IC149.6(C:O) IC149.8(D:O) IC149.9(D:I) IC149.10(E:O) IC149.11(E:I) IC149.12(F:O) IC149.13(F:I) IC150.3(B:I0) IC150.4(B:I1) IC150.5(B:I2) IC150.6(B:O) IC150.8(C:O) IC150.9(C:I0) IC150.10(C:I1) IC150.11(C:I2) IC151.3(B:I0) IC151.4(B:I1) IC151.5(B:I2) IC151.6(B:O) IC151.8(C:O) IC151.9(C:I0) IC151.10(C:I1) IC151.11(C:I2) IC152.1(A:I0) IC152.2(A:I1) IC152.3(A:O) IC152.4(B:I0) IC152.5(B:I1) IC152.6(B:O) IC152.11(D:O) IC152.12(D:I0) IC152.13(D:I1) IC153.11(CLK) IC155.3(1C3) IC155.13(2C3) IC156.3(1C3) IC156.13(2C3) IC157.3(B:I0) IC157.4(B:I1) IC157.5(B:I2) IC157.6(B:O) IC157.8(C:O) IC157.9(C:I0) IC157.10(C:I1) IC157.11(C:I2) IC158.3(B:I0) IC158.4(B:I1) IC158.5(B:I2) IC158.6(B:O) IC158.8(C:O) IC158.9(C:I0) IC158.10(C:I1) IC158.11(C:I2) IC159.6(W) IC159.7(G) IC159.9(C) IC159.10(B) IC159.11(A) IC159.12(D7) IC159.13(D6) IC160.6(W) IC160.7(G) IC160.9(C) IC160.10(B) IC160.11(A) IC160.12(D7) IC160.13(D6) IC161.4(B:I0) IC161.5(B:I1) IC161.6(B:O) IC161.8(C:O) IC161.9(C:I0) IC161.10(C:I1) IC161.11(D:O) IC161.12(D:I0) IC161.13(D:I1) IC163.6(A:!Q) IC163.8(B:!Q) IC163.9(B:Q) IC163.10(B:PRE) IC163.11(B:CLK) IC163.12(B:D) IC163.13(B:CLR) IC164.6(A:!Q) IC164.8(B:!Q) IC164.9(B:Q) IC164.10(B:PRE) IC164.11(B:CLK) IC164.12(B:D) IC164.13(B:CLR) IC165.11(CLK) IC166.11(CLK) IC167.5(2A) IC167.6(2B) IC167.7(2Y) IC167.9(3Y) IC167.10(3B) IC167.11(3A) IC167.12(4Y) IC167.13(4B) IC167.14(4A) IC168.6(A:!Q) IC168.8(B:!Q) IC168.9(B:Q) IC168.10(B:PRE) IC168.11(B:CLK) IC168.12(B:D) IC168.13(B:CLR) IC169.5(2Q) IC169.6(3Q) IC169.9(4Q) IC169.11(CLK) IC169.12(5Q) IC169.15(6Q) IC169.16(7Q) IC170.1(A:I0) IC170.2(A:I1) IC170.3(A:O) IC170.8(C:O) IC170.9(C:I0) IC170.10(C:I1) IC170.11(D:O) IC170.12(D:I0) IC170.13(D:I1) IC171.12(Y7) IC171.13(Y6) IC171.14(Y5) IC171.15(Y4) IC171.16(Y3) IC171.17(Y2) IC172.6(W) IC172.7(G) IC172.9(C) IC172.10(B) IC172.11(A) IC172.12(D7) IC172.13(D6) IC173.11(CLK) IC174.6(A:!Q) IC174.8(B:!Q) IC174.9(B:Q) IC174.10(B:PRE) IC174.11(B:CLK) IC174.12(B:D) IC174.13(B:CLR) IC175.1(A:I0) IC175.2(A:I1) IC175.3(A:O) IC175.8(C:O) IC175.9(C:I0) IC175.10(C:I1) IC175.11(D:O) IC175.12(D:I0) IC175.13(D:I1) IC176.3(B:Y4) IC176.5(B:Y3) IC176.7(B:Y2) IC176.9(B:Y1) IC176.11(B:A1) IC176.13(B:A2) IC176.15(B:A3) IC176.17(B:A4) IC176.19(B:G) IC177.1(A:I0) IC177.2(A:I1) IC177.3(A:O) IC177.8(C:O) IC177.9(C:I0) IC177.10(C:I1) IC177.11(D:O) IC177.12(D:I0) IC177.13(D:I1) IC178.3(B:Y4) IC178.5(B:Y3) IC178.7(B:Y2) IC178.9(B:Y1) IC178.11(B:A1) IC178.13(B:A2) IC178.15(B:A3) IC178.17(B:A4) IC178.19(B:G) IC179.3(B:Y4) IC179.5(B:Y3) IC179.7(B:Y2) IC179.9(B:Y1) IC179.11(B:A1) IC179.13(B:A2) IC179.15(B:A3) IC179.17(B:A4) IC179.19(B:G) IC180.11(CLK) IC181.3(B:Y4) IC181.5(B:Y3) IC181.7(B:Y2) IC181.9(B:Y1) IC181.11(B:A1) IC181.13(B:A2) IC181.15(B:A3) IC181.17(B:A4) IC181.19(B:G) IC182.3(B:Y4) IC182.5(B:Y3) IC182.7(B:Y2) IC182.9(B:Y1) IC182.11(B:A1) IC182.13(B:A2) IC182.15(B:A3) IC182.17(B:A4) IC182.19(B:G) IC183.3(B:Y4) IC183.5(B:Y3) IC183.7(B:Y2) IC183.9(B:Y1) IC183.11(B:A1) IC183.13(B:A2) IC183.15(B:A3) IC183.17(B:A4) IC183.19(B:G) IC184.11(CLK) IC185.11(CLK) IC186.6(W) IC186.7(G) IC186.9(C) IC186.10(B) IC186.11(A) IC186.12(D7) IC186.13(D6) IC187.6(A:!Q) IC187.8(B:!Q) IC187.9(B:Q) IC187.10(B:PRE) IC187.11(B:CLK) IC187.12(B:D) IC187.13(B:CLR) IC188.6(A:!Q) IC188.8(B:!Q) IC188.9(B:Q) IC188.10(B:PRE) IC188.11(B:CLK) IC188.12(B:D) IC188.13(B:CLR) IC189.4(2D) IC189.7(3D) IC189.8(4D) IC189.13(5D) IC189.14(6D) IC189.17(7D) IC190.1(A:I0) IC190.2(A:I1) IC190.3(A:O) IC190.4(B:I0) IC190.5(B:I1) IC190.6(B:O) IC190.11(D:O) IC190.12(D:I0) IC190.13(D:I1) IC191.3(B:I0) IC191.4(B:I1) IC191.5(B:I2) IC191.6(B:O) IC191.8(C:O) IC191.9(C:I0) IC191.10(C:I1) IC191.11(C:I2) IC192.1(A:I0) IC192.2(A:I1) IC192.3(A:O) IC192.8(C:O) IC192.9(C:I0) IC192.10(C:I1) IC192.11(D:O) IC192.12(D:I0) IC192.13(D:I1) IC193.1(A:I0) IC193.2(A:I1) IC193.3(A:O) IC193.8(C:O) IC193.9(C:I0) IC193.10(C:I1) IC193.11(D:O) IC193.12(D:I0) IC193.13(D:I1) IC194.1(A:I0) IC194.2(A:I1) IC194.3(A:O) IC194.8(C:O) IC194.9(C:I0) IC194.10(C:I1) IC194.11(D:O) IC194.12(D:I0) IC194.13(D:I1) IC195.4(B:I0) IC195.5(B:I1) IC195.6(B:O) IC195.8(C:O) IC195.9(C:I0) IC195.10(C:I1) IC195.11(D:O) IC195.12(D:I0) IC195.13(D:I1) IC196.1(A:I) IC196.2(A:O) IC196.5(C:I) IC196.6(C:O) IC196.8(D:O) IC196.9(D:I) IC196.10(E:O) IC196.11(E:I) IC196.12(F:O) IC196.13(F:I) IC197.4(B:I0) IC197.6(B:O) IC197.8(B:I1) IC197.9(B:I2) IC197.10(B:I3) IC197.11(B:I4) IC198.3(B:I) IC198.4(B:O) IC198.5(C:I) IC198.6(C:O) IC198.8(D:O) IC198.9(D:I) IC198.10(E:O) IC198.11(E:I) IC198.12(F:O) IC198.13(F:I) IC199.4(B:I0) IC199.6(B:O) IC199.8(B:I1) IC199.9(B:I2) IC199.10(B:I3) IC199.11(B:I4) IC200.1(A:I0) IC200.2(A:I1) IC200.3(A:O) IC200.8(C:O) IC200.9(C:I0) IC200.10(C:I1) IC200.11(D:O) IC200.12(D:I0) IC200.13(D:I1) IC201.1(A:I0) IC201.2(A:I1) IC201.3(A:O) IC201.4(B:I0) IC201.5(B:I1) IC201.6(B:O) IC201.11(D:O) IC201.12(D:I0) IC201.13(D:I1) IC202.11(CLK) IC203.1(A:I0) IC203.2(A:I1) IC203.3(A:O) IC203.4(B:I0) IC203.5(B:I1) IC203.6(B:O) IC203.11(D:O) IC203.12(D:I0) IC203.13(D:I1) IC204.6(A:!Q) IC204.8(B:!Q) IC204.9(B:Q) IC204.10(B:PRE) IC204.11(B:CLK) IC204.12(B:D) IC204.13(B:CLR) IC205.11(CLK) IC206.1(A:I0) IC206.2(A:I1) IC206.3(A:O) IC206.4(B:I0) IC206.5(B:I1) IC206.6(B:O) IC206.11(D:O) IC206.12(D:I0) IC206.13(D:I1) IC207.4(B:I0) IC207.5(B:I1) IC207.6(B:O) IC207.8(C:O) IC207.9(C:I0) IC207.10(C:I1) IC207.11(D:O) IC207.12(D:I0) IC207.13(D:I1) IC208.1(1G) IC208.9(2Y) IC208.10(2C0) IC208.11(2C1) IC208.12(2C2) IC208.13(2C3) IC208.15(2G) IC209.1(A:I0) IC209.2(A:I1) IC209.3(A:O) IC209.8(C:O) IC209.9(C:I0) IC209.10(C:I1) IC209.11(D:O) IC209.12(D:I0) IC209.13(D:I1) IC210.12(Y7) IC210.13(Y6) IC210.14(Y5) IC210.15(Y4) IC210.16(Y3) IC210.17(Y2) IC211.3(B:Y4) IC211.5(B:Y3) IC211.7(B:Y2) IC211.9(B:Y1) IC211.11(B:A1) IC211.13(B:A2) IC211.15(B:A3) IC211.17(B:A4) IC211.19(B:G) IC212.3(B:Y4) IC212.5(B:Y3) IC212.7(B:Y2) IC212.9(B:Y1) IC212.11(B:A1) IC212.13(B:A2) IC212.15(B:A3) IC212.17(B:A4) IC212.19(B:G) IC213.3(B:Y4) IC213.5(B:Y3) IC213.7(B:Y2) IC213.9(B:Y1) IC213.11(B:A1) IC213.13(B:A2) IC213.15(B:A3) IC213.17(B:A4) IC213.19(B:G) IC214.3(B:Y4) IC214.5(B:Y3) IC214.7(B:Y2) IC214.9(B:Y1) IC214.11(B:A1) IC214.13(B:A2) IC214.15(B:A3) IC214.17(B:A4) IC214.19(B:G) IC215.12(Y7) IC215.13(Y6) IC215.14(Y5) IC215.15(Y4) IC215.16(Y3) IC215.17(Y2) IC216.1(G) IC216.11(CLK) IC217.11(CLK) IC218.4(B:I0) IC218.5(B:I1) IC218.6(B:O) IC218.8(C:O) IC218.9(C:I0) IC218.10(C:I1) IC218.11(D:O) IC218.12(D:I0) IC218.13(D:I1) IC219.4(B:I0) IC219.5(B:I1) IC219.6(B:O) IC219.8(C:O) IC219.9(C:I0) IC219.10(C:I1) IC219.11(D:O) IC219.12(D:I0) IC219.13(D:I1) IC220.4(B:I0) IC220.5(B:I1) IC220.6(B:O) IC220.8(C:O) IC220.9(C:I0) IC220.10(C:I1) IC220.11(D:O) IC220.12(D:I0) IC220.13(D:I1) IC221.6(A:!Q) IC221.8(B:!Q) IC221.9(B:Q) IC221.10(B:PRE) IC221.11(B:CLK) IC221.12(B:D) IC221.13(B:CLR) IC223.4(B:I0) IC223.5(B:I1) IC223.6(B:O) IC223.8(C:O) IC223.9(C:I0) IC223.10(C:I1) IC223.11(D:O) IC223.12(D:I0) IC223.13(D:I1) IC224.4(B:I0) IC224.5(B:I1) IC224.6(B:O) IC224.8(C:O) IC224.9(C:I0) IC224.10(C:I1) IC224.11(D:O) IC224.12(D:I0) IC224.13(D:I1) IC225.4(B:I0) IC225.5(B:I1) IC225.6(B:O) IC225.8(C:O) IC225.9(C:I0) IC225.10(C:I1) IC225.11(D:O) IC225.12(D:I0) IC225.13(D:I1) IC227.11(CLK) IC228.1(A:I0) IC228.2(A:I1) IC228.3(A:O) IC228.4(B:I0) IC228.5(B:I1) IC228.6(B:O) IC228.11(D:O) IC228.12(D:I0) IC228.13(D:I1) IC229.3(B:Y4) IC229.5(B:Y3) IC229.7(B:Y2) IC229.9(B:Y1) IC229.11(B:A1) IC229.13(B:A2) IC229.15(B:A3) IC229.17(B:A4) IC229.19(B:G) IC230.3(B:Y4) IC230.5(B:Y3) IC230.7(B:Y2) IC230.9(B:Y1) IC230.11(B:A1) IC230.13(B:A2) IC230.15(B:A3) IC230.17(B:A4) IC230.19(B:G) IC231.3(B:Y4) IC231.5(B:Y3) IC231.7(B:Y2) IC231.9(B:Y1) IC231.11(B:A1) IC231.13(B:A2) IC231.15(B:A3) IC231.17(B:A4) IC231.19(B:G) IC232.3(B:Y4) IC232.5(B:Y3) IC232.7(B:Y2) IC232.9(B:Y1) IC232.11(B:A1) IC232.13(B:A2) IC232.15(B:A3) IC232.17(B:A4) IC232.19(B:G) IC233.11(CLK) IC234.11(CLK) IC235.3(B:Y4) IC235.5(B:Y3) IC235.7(B:Y2) IC235.9(B:Y1) IC235.11(B:A1) IC235.13(B:A2) IC235.15(B:A3) IC235.17(B:A4) IC235.19(B:G) IC236.3(B:Y4) IC236.5(B:Y3) IC236.7(B:Y2) IC236.9(B:Y1) IC236.11(B:A1) IC236.13(B:A2) IC236.15(B:A3) IC236.17(B:A4) IC236.19(B:G) IC237.3(B:Y4) IC237.5(B:Y3) IC237.7(B:Y2) IC237.9(B:Y1) IC237.11(B:A1) IC237.13(B:A2) IC237.15(B:A3) IC237.17(B:A4) IC237.19(B:G) IC238.3(B:Y4) IC238.5(B:Y3) IC238.7(B:Y2) IC238.9(B:Y1) IC238.11(B:A1) IC238.13(B:A2) IC238.15(B:A3) IC238.17(B:A4) IC238.19(B:G) IC239.11(CLK) IC240.11(CLK) IC241.1(1G) IC241.9(2Y) IC241.10(2C0) IC241.11(2C1) IC241.12(2C2) IC241.13(2C3) IC241.15(2G) IC242.1(A:I0) IC242.2(A:I1) IC242.3(A:O) IC242.4(B:I0) IC242.5(B:I1) IC242.6(B:O) IC242.11(D:O) IC242.12(D:I0) IC242.13(D:I1) IC243.1(1G) IC243.9(2Y) IC243.10(2C0) IC243.11(2C1) IC243.12(2C2) IC243.13(2C3) IC243.15(2G) IC244.1(A:G) IC244.2(A:A1) IC244.4(A:A2) IC244.5(B:Y3) IC244.6(A:A3) IC244.7(B:Y2) IC244.8(A:A4) IC244.12(A:Y4) IC244.14(A:Y3) IC244.16(A:Y2) IC244.18(A:Y1) IC246.11(CLK) IC247.1(A:G) IC247.2(A:A1) IC247.4(A:A2) IC247.5(B:Y3) IC247.6(A:A3) IC247.7(B:Y2) IC247.8(A:A4) IC247.12(A:Y4) IC247.14(A:Y3) IC247.16(A:Y2) IC247.18(A:Y1) IC250.1(A:I0) IC250.2(A:I1) IC250.3(A:O) IC250.8(C:O) IC250.9(C:I0) IC250.10(C:I1) IC250.11(D:O) IC250.12(D:I0) IC250.13(D:I1) IC251.11(CLK) IC252.12(Y7) IC252.13(Y6) IC252.14(Y5) IC252.15(Y4) IC252.16(Y3) IC252.17(Y2) IC253.12(Y7) IC253.13(Y6) IC253.14(Y5) IC253.15(Y4) IC253.16(Y3) IC253.17(Y2) IC254.11(CLK) IC255.1(1G) IC255.9(2Y) IC255.10(2C0) IC255.11(2C1) IC255.12(2C2) IC255.13(2C3) IC255.15(2G) IC256.1(1G) IC256.9(2Y) IC256.10(2C0) IC256.11(2C1) IC256.12(2C2) IC256.13(2C3) IC256.15(2G) IC257.15(G) IC259.12(Y7) IC259.13(Y6) IC259.14(Y5) IC259.15(Y4) IC259.16(Y3) IC259.17(Y2) IC260.12(Y7) IC260.13(Y6) IC260.14(Y5) IC260.15(Y4) IC260.16(Y3) IC260.17(Y2) IC261.11(CLK) IC262.11(CLK) IC263.12(Y7) IC263.13(Y6) IC263.14(Y5) IC263.15(Y4) IC263.16(Y3) IC263.17(Y2) IC264.12(Y7) IC264.13(Y6) IC264.14(Y5) IC264.15(Y4) IC264.16(Y3) IC264.17(Y2) IC265.11(CLK) IC266.12(Y7) IC266.13(Y6) IC266.14(Y5) IC266.15(Y4) IC266.16(Y3) IC266.17(Y2) IC267.12(Y7) IC267.13(Y6) IC267.14(Y5) IC267.15(Y4) IC267.16(Y3) IC267.17(Y2) IC269.4(B:I0) IC269.5(B:I1) IC269.6(B:O) IC269.8(C:O) IC269.9(C:I0) IC269.10(C:I1) IC269.11(D:O) IC269.12(D:I0) IC269.13(D:I1) IC270.1(A:I) IC270.2(A:O) IC270.5(C:I) IC270.6(C:O) IC270.8(D:O) IC270.9(D:I) IC270.10(E:O) IC270.11(E:I) IC270.12(F:O) IC270.13(F:I) IC271.1(A:I) IC271.2(A:O) IC271.5(C:I) IC271.6(C:O) IC271.8(D:O) IC271.9(D:I) IC271.10(E:O) IC271.11(E:I) IC271.12(F:O) IC271.13(F:I) IC272.1(!A!/B) IC277.1(!A!/B) IC287.9(C4) IC288.3(B:Y4) IC288.5(B:Y3) IC288.7(B:Y2) IC288.9(B:Y1) IC288.11(B:A1) IC288.13(B:A2) IC288.15(B:A3) IC288.17(B:A4) IC288.19(B:G) IC289.3(B:Y4) IC289.5(B:Y3) IC289.7(B:Y2) IC289.9(B:Y1) IC289.11(B:A1) IC289.13(B:A2) IC289.15(B:A3) IC289.17(B:A4) IC289.19(B:G) IC290.3(B:Y4) IC290.5(B:Y3) IC290.7(B:Y2) IC290.9(B:Y1) IC290.11(B:A1) IC290.13(B:A2) IC290.15(B:A3) IC290.17(B:A4) IC290.19(B:G) IC291.3(B:Y4) IC291.5(B:Y3) IC291.7(B:Y2) IC291.9(B:Y1) IC291.11(B:A1) IC291.13(B:A2) IC291.15(B:A3) IC291.17(B:A4) IC291.19(B:G) IC292.3(B:Y4) IC292.5(B:Y3) IC292.7(B:Y2) IC292.9(B:Y1) IC292.11(B:A1) IC292.13(B:A2) IC292.15(B:A3) IC292.17(B:A4) IC292.19(B:G) IC293.3(B:Y4) IC293.5(B:Y3) IC293.7(B:Y2) IC293.9(B:Y1) IC293.11(B:A1) IC293.13(B:A2) IC293.15(B:A3) IC293.17(B:A4) IC293.19(B:G) IC294.3(B:Y4) IC294.5(B:Y3) IC294.7(B:Y2) IC294.9(B:Y1) IC294.11(B:A1) IC294.13(B:A2) IC294.15(B:A3) IC294.17(B:A4) IC294.19(B:G) IC295.3(B:Y4) IC295.5(B:Y3) IC295.7(B:Y2) IC295.9(B:Y1) IC295.11(B:A1) IC295.13(B:A2) IC295.15(B:A3) IC295.17(B:A4) IC295.19(B:G) IC296.11(CLK) IC297.3(B:Y4) IC297.5(B:Y3) IC297.7(B:Y2) IC297.9(B:Y1) IC297.11(B:A1) IC297.13(B:A2) IC297.15(B:A3) IC297.17(B:A4) IC297.19(B:G) IC298.3(B:Y4) IC298.5(B:Y3) IC298.7(B:Y2) IC298.9(B:Y1) IC298.11(B:A1) IC298.13(B:A2) IC298.15(B:A3) IC298.17(B:A4) IC298.19(B:G) IC299.3(B:Y4) IC299.5(B:Y3) IC299.7(B:Y2) IC299.9(B:Y1) IC299.11(B:A1) IC299.13(B:A2) IC299.15(B:A3) IC299.17(B:A4) IC299.19(B:G) IC300.3(B:Y4) IC300.5(B:Y3) IC300.7(B:Y2) IC300.9(B:Y1) IC300.11(B:A1) IC300.13(B:A2) IC300.15(B:A3) IC300.17(B:A4) IC300.19(B:G) IC301.11(CLK) IC302.12(Y7) IC302.13(Y6) IC302.14(Y5) IC302.15(Y4) IC302.16(Y3) IC302.17(Y2) IC302.18(Y1) IC303.12(Y7) IC303.13(Y6) IC303.14(Y5) IC303.15(Y4) IC303.16(Y3) IC303.17(Y2) RN4.4 RN4.5 RN4.6 RN4.7 RN4.8 RN4.9 RN4.10 RN4.11 RN4.12 RN4.13 S2.1(O) S4.1(O) SW3.8 U$1.28(VCC) U$2.28(VCC) U$3.28(VCC) U$4.28(VCC) U$5.28(VCC) U$6.28(VCC) U$7.28(VCC) U$8.28(VCC) U$9.28(VCC) U$10.1(A14) U$10.2(A12) U$10.3(A7) U$10.4(A6) U$10.5(A5) U$10.6(A4) U$10.7(A3) U$10.8(A2) U$10.9(A1) U$10.10(A0) U$10.14(GND) U$10.20(/CE) U$10.21(A10) U$10.22(/OE) U$10.23(A11) U$10.24(A9) U$10.25(A8) U$10.26(A13) U$10.27(/WE) U$10.28(VCC) U$11.1(A14) U$11.2(A12) U$11.3(A7) U$11.4(A6) U$11.5(A5) U$11.6(A4) U$11.7(A3) U$11.8(A2) U$11.9(A1) U$11.10(A0) U$11.14(GND) U$11.20(/CE) U$11.21(A10) U$11.22(/OE) U$11.23(A11) U$11.24(A9) U$11.25(A8) U$11.26(A13) U$11.27(/WE) U$11.28(VCC) U$12.1(A14) U$12.2(A12) U$12.3(A7) U$12.4(A6) U$12.5(A5) U$12.6(A4) U$12.7(A3) U$12.8(A2) U$12.9(A1) U$12.10(A0) U$12.14(GND) U$12.20(/CE) U$12.21(A10) U$12.22(/OE) U$12.23(A11) U$12.24(A9) U$12.25(A8) U$12.26(A13) U$12.27(/WE) U$12.28(VCC)

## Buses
XBUS[0..7]
ZBUS[0..7]
YBUS[0..7]
AD[0..19]
MDR_IN_BUS[0..7]
U_AD[0..15]
DATA[0..7]

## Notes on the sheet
- The codename DreamCatcher homemade 8/16bit CPU/Minicomputer
  Conceived & designed by Paulo Constantino - pconst167@gmail.com
  
  The purpose of designing this CPU/Minicomputer was manyfold. 
  Firstly it will be aimed at students who are looking for practice in 
  building computer CPU's and systems. 
  Seconly, it will be connected to the internet by myself (and maybe others who will follow) 
  and used to host a bulletin-board like system whereby enthusiasts and students can log-on, 
  download files, schematics, use forums, chat, play games, and many other activities. 
  This should inspire people to study and build it, if they see that it works well. 
  And lastly, designing and building computers is just pure ecstasy!!
  
  Shareware - Share with passion!!
  
  This file is probably a .png image. For the original Eagle schematics, ask by e-mail!
- DMA CAN ONLY HAPPEN IF WE ARE NOT TRAPPING.
- SYNCHRONIZED INTERRUPT INPUTS
- TRAP
  INT_REQ_0
  INT_REQ_1
  INT_REQ_2
  INT_REQ_3
  INT_REQ_4
  INT_REQ_5
  INT_REQ_6
- R_SHIFT_L
- SINGLE STEP CLOCK
- fast clock
- slow clock
- IF A TRAP HAPPENS, THEN NEITHER MASKABLE INTERRUPTS
  NOR TRAPS ARE ALLOWED TO HAPPEN.
  
  THIS IS DICTATED BY THE TRAP_ENABLE SIGNAL
- R_SHIFT_H
- the encoded bits start at position 3 in the byte. 
  this is so it's easier to just transfer this to PC and 
  have it become the interrupt vector in memory.
  
  so each interrupt spans 8 bytes in memory.
  
  00000000 = int_0
  00001000 = int_1
  00010000 = int_2
  00011000 = int_3
  etc
- IMMX
- TDR0_L
- TDR0_H
- TDR1_L
- U-ADDRESS MUX
- TDR1_H
- ADDRESS & DATA BUSES NEED PULL DOWN RESISTORS 
  BECAUSE THE CPU BUS OUTPUTS HAVE 
  244'S WHICH ARE CLOSED MOST OF THE TIME.
- LOW
- CS_L
- CS_H
- MASK_FLAGS
- OFFSET(6)
- DS_L
- IR_L
- HIGH
- DS_H
- AL
- Z BUS
- PC_L
- U-CODE ROMS
- U-ADDRESS
- U-CODE FF'S
- SS_L
- IR_H
- AH
- LOW | PC_H
- MARL
- SS_H
- LOW
- ADDER
- BL
- HIGH
- SP_L
- ES_L
- BH
- ADDER
- MARH
- MAR is tri-stated when in programming or DMA mode. | SP_H
- ES_H
- programming mode signal goes here to tell MAR to go tristate
- AUX_FLAGS
- CL
- SI_L
- BP_L
- CH
- if type = branch, and condition = false, then next = +1
- HIGH
- SI_H
- BP_H
- DL
- Z BUS
- DI_L
- FLAGS REGISTER
- DH
- DI_H
- CARRY IN MUX
- U_FLAGS
- BUS GOING INTO MDR INPUTS
- X BUS
- CONDITION SOURCE
  PROGRAMMER'S FLAGS 
  OR
  U_CODE FLAGS
- MDRL_L
- ZF | DATA BUS
- CF / LTU
- MDRL_H
- SF | MDR MUX | BUS GOING INTO MDR INPUTS
- IMMY
- OF
- PF
- ALU
- LT
  LTE
  ~LT = GTE
  ~LTE + GT
- alu_mode removed. OF is undefined if alu in logic mode anyway. | alu_op == add
- DATA BUS
- SERIES TERMINATION ~80 ohm
- ALU_OP == SUB
- MDRH_L
- MDRH_H
- DATA BUS
- TDR0_L
- IMMY
- TDR0_H
- FROM MICROCODE
- TDR1_L
- TDR1_H

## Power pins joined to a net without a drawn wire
GND: IC1.10(GND) IC2.10(GND) IC3.10(GND) IC4.10(GND) IC5.10(GND) IC6.10(GND) IC7.10(GND) IC8.7(P:GND) IC9.10(GND) IC10.10(P:GND) IC11.10(P:GND) IC12.10(P:GND) IC13.10(P:GND) IC14.12(GND) IC15.12(GND) IC16.10(GND) IC17.10(GND) IC18.7(P:GND) IC19.10(GND) IC20.8(GND) IC21.10(GND) IC22.8(GND) IC23.8(GND) IC24.10(P:GND) IC25.10(P:GND) IC26.10(P:GND) IC27.10(P:GND) IC28.10(GND) IC30.10(P:GND) IC31.10(P:GND) IC32.10(GND) IC33.10(GND) IC34.8(GND) IC35.8(GND) IC36.8(GND) IC37.8(GND) IC38.8(GND) IC39.7(P:GND) IC40.8(GND) IC41.8(GND) IC42.7(P:GND) IC43.7(P:GND) IC44.7(P:GND) IC45.7(P:GND) IC46.7(P:GND) IC47.7(P:GND) IC48.10(GND) IC49.8(GND) IC50.8(GND) IC51.8(GND) IC52.8(GND) IC53.8(GND) IC54.7(P:GND) IC55.8(GND) IC56.8(GND) IC57.7(P:GND) IC58.7(P:GND) IC59.7(P:GND) IC60.10(GND) IC61.10(GND) IC62.10(GND) IC63.8(GND) IC64.7(P:GND) IC65.7(P:GND) IC66.7(P:GND) IC67.7(P:GND) IC68.8(GND) IC69.10(P:GND) IC70.8(GND) IC71.8(GND) IC72.7(P:GND) IC73.8(GND) IC74.7(P:GND) IC75.10(GND) IC76.10(GND) IC77.10(GND) IC78.10(GND) IC79.10(GND) IC80.7(P:GND) IC81.7(P:GND) IC82.10(GND) IC83.7(P:GND) IC84.7(P:GND) IC85.7(P:GND) IC86.10(GND) IC87.8(P:GND) IC88.10(GND) IC89.10(P:GND) IC90.10(P:GND) IC91.10(P:GND) IC92.10(P:GND) IC93.10(GND) IC94.8(GND) IC95.8(GND) IC96.8(GND) IC97.8(GND) IC98.10(GND) IC99.10(GND) IC100.10(GND) IC101.10(GND) IC102.10(GND) IC103.10(GND) IC104.10(GND) IC105.10(P:GND) IC106.10(P:GND) IC107.10(P:GND) IC108.10(P:GND) IC109.10(P:GND) IC110.10(P:GND) IC111.10(P:GND) IC112.10(P:GND) IC113.10(GND) IC114.10(GND) IC115.10(GND) IC116.10(GND) IC117.10(GND) IC118.10(GND) IC119.7(P:GND) IC120.7(P:GND) IC121.8(GND) IC122.10(GND) IC123.10(GND) IC124.7(P:GND) IC125.10(GND) IC126.10(GND) IC127.7(P:GND) IC128.8(GND) IC129.8(GND) IC130.7(P:GND) IC131.7(P:GND) IC132.7(P:GND) IC133.7(P:GND) IC134.10(GND) IC135.10(GND) IC136.10(GND) IC137.10(GND) IC138.7(P:GND) IC139.8(GND) IC140.10(GND) IC141.7(P:GND) IC142.8(GND) IC143.7(P:GND) IC144.8(GND) IC145.10(GND) IC146.10(GND) IC147.7(P:GND) IC148.7(P:GND) IC149.7(P:GND) IC150.7(P:GND) IC151.7(P:GND) IC152.7(P:GND) IC153.10(GND) IC154.10(GND) IC155.8(GND) IC156.8(GND) IC157.7(P:GND) IC158.7(P:GND) IC159.8(GND) IC160.8(GND) IC161.7(P:GND) IC162.10(GND) IC163.7(P:GND) IC164.7(P:GND) IC165.10(GND) IC166.10(GND) IC167.8(GND) IC168.7(P:GND) IC169.10(GND) IC170.7(P:GND) IC171.10(GND) IC172.8(GND) IC173.10(GND) IC174.7(P:GND) IC175.7(P:GND) IC176.10(P:GND) IC177.7(P:GND) IC178.10(P:GND) IC179.10(P:GND) IC180.10(GND) IC181.10(P:GND) IC182.10(P:GND) IC183.10(P:GND) IC184.10(GND) IC185.10(GND) IC186.8(GND) IC187.7(P:GND) IC188.7(P:GND) IC189.10(GND) IC190.7(P:GND) IC191.7(P:GND) IC192.7(P:GND) IC193.7(P:GND) IC194.7(P:GND) IC195.7(P:GND) IC196.7(P:GND) IC197.7(P:GND) IC198.7(P:GND) IC199.7(P:GND) IC200.7(P:GND) IC201.7(P:GND) IC202.10(GND) IC203.7(P:GND) IC204.7(P:GND) IC205.10(GND) IC206.7(P:GND) IC207.7(P:GND) IC208.8(GND) IC209.7(P:GND) IC210.10(GND) IC211.10(P:GND) IC212.10(P:GND) IC213.10(P:GND) IC214.10(P:GND) IC215.10(GND) IC216.10(GND) IC217.10(GND) IC218.7(P:GND) IC219.7(P:GND) IC220.7(P:GND) IC221.7(P:GND) IC222.8(GND) IC223.7(P:GND) IC224.7(P:GND) IC225.7(P:GND) IC226.8(GND) IC227.10(GND) IC228.7(P:GND) IC229.10(P:GND) IC230.10(P:GND) IC231.10(P:GND) IC232.10(P:GND) IC233.10(GND) IC234.10(GND) IC235.10(P:GND) IC236.10(P:GND) IC237.10(P:GND) IC238.10(P:GND) IC239.10(GND) IC240.10(GND) IC241.8(GND) IC242.7(P:GND) IC243.8(GND) IC244.10(P:GND) IC245.10(GND) IC246.10(GND) IC247.10(P:GND) IC248.8(GND) IC249.8(GND) IC250.7(P:GND) IC251.10(GND) IC252.10(GND) IC253.10(GND) IC254.10(GND) IC255.8(GND) IC256.8(GND) IC257.8(GND) IC258.8(GND) IC259.10(GND) IC260.10(GND) IC261.10(GND) IC262.10(GND) IC263.10(GND) IC264.10(GND) IC265.10(GND) IC266.10(GND) IC267.10(GND) IC268.8(GND) IC269.7(P:GND) IC270.7(P:GND) IC271.7(P:GND) IC272.8(GND) IC273.8(GND) IC274.8(GND) IC275.8(GND) IC276.8(GND) IC277.8(GND) IC278.8(GND) IC279.8(GND) IC280.8(GND) IC281.8(GND) IC282.8(GND) IC283.8(GND) IC284.8(GND) IC285.8(GND) IC286.8(GND) IC287.8(GND) IC288.10(P:GND) IC289.10(P:GND) IC290.10(P:GND) IC291.10(P:GND) IC292.10(P:GND) IC293.10(P:GND) IC294.10(P:GND) IC295.10(P:GND) IC296.10(GND) IC297.10(P:GND) IC298.10(P:GND) IC299.10(P:GND) IC300.10(P:GND) IC301.10(GND) IC302.10(GND) IC303.10(GND)
VCC: IC1.20(VCC) IC2.20(VCC) IC3.20(VCC) IC4.20(VCC) IC5.20(VCC) IC6.20(VCC) IC7.20(VCC) IC8.14(P:VCC) IC9.20(VCC) IC10.20(P:VCC) IC11.20(P:VCC) IC12.20(P:VCC) IC13.20(P:VCC) IC14.24(VCC) IC15.24(VCC) IC16.20(VCC) IC17.20(VCC) IC18.14(P:VCC) IC19.20(VCC) IC20.16(VCC) IC21.20(VCC) IC22.16(VCC) IC23.16(VCC) IC24.20(P:VCC) IC25.20(P:VCC) IC26.20(P:VCC) IC27.20(P:VCC) IC28.20(VCC) IC30.20(P:VCC) IC31.20(P:VCC) IC32.20(VCC) IC33.20(VCC) IC34.16(VCC) IC35.16(VCC) IC36.16(VCC) IC37.16(VCC) IC38.16(VCC) IC39.14(P:VCC) IC40.16(VCC) IC41.16(VCC) IC42.14(P:VCC) IC43.14(P:VCC) IC44.14(P:VCC) IC45.14(P:VCC) IC46.14(P:VCC) IC47.14(P:VCC) IC48.20(VCC) IC49.16(VCC) IC50.16(VCC) IC51.16(VCC) IC52.16(VCC) IC53.16(VCC) IC54.14(P:VCC) IC55.16(VCC) IC56.16(VCC) IC57.14(P:VCC) IC58.14(P:VCC) IC59.14(P:VCC) IC60.20(VCC) IC61.20(VCC) IC62.20(VCC) IC63.16(VCC) IC64.14(P:VCC) IC65.14(P:VCC) IC66.14(P:VCC) IC67.14(P:VCC) IC68.16(VCC) IC69.20(P:VCC) IC70.16(VCC) IC71.16(VCC) IC72.14(P:VCC) IC73.16(VCC) IC74.14(P:VCC) IC75.20(VCC) IC76.20(VCC) IC77.20(VCC) IC78.20(VCC) IC79.20(VCC) IC80.14(P:VCC) IC81.14(P:VCC) IC82.20(VCC) IC83.14(P:VCC) IC84.14(P:VCC) IC85.14(P:VCC) IC86.20(VCC) IC87.16(P:VCC) IC88.20(VCC) IC89.20(P:VCC) IC90.20(P:VCC) IC91.20(P:VCC) IC92.20(P:VCC) IC93.20(VCC) IC94.16(VCC) IC95.16(VCC) IC96.16(VCC) IC97.16(VCC) IC98.20(VCC) IC99.20(VCC) IC100.20(VCC) IC101.20(VCC) IC102.20(VCC) IC103.20(VCC) IC104.20(VCC) IC105.20(P:VCC) IC106.20(P:VCC) IC107.20(P:VCC) IC108.20(P:VCC) IC109.20(P:VCC) IC110.20(P:VCC) IC111.20(P:VCC) IC112.20(P:VCC) IC113.20(VCC) IC114.20(VCC) IC115.20(VCC) IC116.20(VCC) IC117.20(VCC) IC118.20(VCC) IC119.14(P:VCC) IC120.14(P:VCC) IC121.16(VCC) IC122.20(VCC) IC123.20(VCC) IC124.14(P:VCC) IC125.20(VCC) IC126.20(VCC) IC127.14(P:VCC) IC128.16(VCC) IC129.16(VCC) IC130.14(P:VCC) IC131.14(P:VCC) IC132.14(P:VCC) IC133.14(P:VCC) IC134.20(VCC) IC135.20(VCC) IC136.20(VCC) IC137.20(VCC) IC138.14(P:VCC) IC139.16(VCC) IC140.20(VCC) IC141.14(P:VCC) IC142.16(VCC) IC143.14(P:VCC) IC144.16(VCC) IC145.20(VCC) IC146.20(VCC) IC147.14(P:VCC) IC148.14(P:VCC) IC149.14(P:VCC) IC150.14(P:VCC) IC151.14(P:VCC) IC152.14(P:VCC) IC153.20(VCC) IC154.20(VCC) IC155.16(VCC) IC156.16(VCC) IC157.14(P:VCC) IC158.14(P:VCC) IC159.16(VCC) IC160.16(VCC) IC161.14(P:VCC) IC162.20(VCC) IC163.14(P:VCC) IC164.14(P:VCC) IC165.20(VCC) IC166.20(VCC) IC167.16(VCC) IC168.14(P:VCC) IC169.20(VCC) IC170.14(P:VCC) IC171.20(VCC) IC172.16(VCC) IC173.20(VCC) IC174.14(P:VCC) IC175.14(P:VCC) IC176.20(P:VCC) IC177.14(P:VCC) IC178.20(P:VCC) IC179.20(P:VCC) IC180.20(VCC) IC181.20(P:VCC) IC182.20(P:VCC) IC183.20(P:VCC) IC184.20(VCC) IC185.20(VCC) IC186.16(VCC) IC187.14(P:VCC) IC188.14(P:VCC) IC189.20(VCC) IC190.14(P:VCC) IC191.14(P:VCC) IC192.14(P:VCC) IC193.14(P:VCC) IC194.14(P:VCC) IC195.14(P:VCC) IC196.14(P:VCC) IC197.14(P:VCC) IC198.14(P:VCC) IC199.14(P:VCC) IC200.14(P:VCC) IC201.14(P:VCC) IC202.20(VCC) IC203.14(P:VCC) IC204.14(P:VCC) IC205.20(VCC) IC206.14(P:VCC) IC207.14(P:VCC) IC208.16(VCC) IC209.14(P:VCC) IC210.20(VCC) IC211.20(P:VCC) IC212.20(P:VCC) IC213.20(P:VCC) IC214.20(P:VCC) IC215.20(VCC) IC216.20(VCC) IC217.20(VCC) IC218.14(P:VCC) IC219.14(P:VCC) IC220.14(P:VCC) IC221.14(P:VCC) IC222.16(VCC) IC223.14(P:VCC) IC224.14(P:VCC) IC225.14(P:VCC) IC226.16(VCC) IC227.20(VCC) IC228.14(P:VCC) IC229.20(P:VCC) IC230.20(P:VCC) IC231.20(P:VCC) IC232.20(P:VCC) IC233.20(VCC) IC234.20(VCC) IC235.20(P:VCC) IC236.20(P:VCC) IC237.20(P:VCC) IC238.20(P:VCC) IC239.20(VCC) IC240.20(VCC) IC241.16(VCC) IC242.14(P:VCC) IC243.16(VCC) IC244.20(P:VCC) IC245.20(VCC) IC246.20(VCC) IC247.20(P:VCC) IC248.16(VCC) IC249.16(VCC) IC250.14(P:VCC) IC251.20(VCC) IC252.20(VCC) IC253.20(VCC) IC254.20(VCC) IC255.16(VCC) IC256.16(VCC) IC257.16(VCC) IC258.16(VCC) IC259.20(VCC) IC260.20(VCC) IC261.20(VCC) IC262.20(VCC) IC263.20(VCC) IC264.20(VCC) IC265.20(VCC) IC266.20(VCC) IC267.20(VCC) IC268.16(VCC) IC269.14(P:VCC) IC270.14(P:VCC) IC271.14(P:VCC) IC272.16(VCC) IC273.16(VCC) IC274.16(VCC) IC275.16(VCC) IC276.16(VCC) IC277.16(VCC) IC278.16(VCC) IC279.16(VCC) IC280.16(VCC) IC281.16(VCC) IC282.16(VCC) IC283.16(VCC) IC284.16(VCC) IC285.16(VCC) IC286.16(VCC) IC287.16(VCC) IC288.20(P:VCC) IC289.20(P:VCC) IC290.20(P:VCC) IC291.20(P:VCC) IC292.20(P:VCC) IC293.20(P:VCC) IC294.20(P:VCC) IC295.20(P:VCC) IC296.20(VCC) IC297.20(P:VCC) IC298.20(P:VCC) IC299.20(P:VCC) IC300.20(P:VCC) IC301.20(VCC) IC302.20(VCC) IC303.20(VCC)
